FUNCTION F_SetStateParams : BOOL;
VAR_INPUT
    nStateRef    :    UDINT;
    rPosition    :    REAL;
    rTolerance: REAL;
    stBeamParams    :    ST_BeamParams;
END_VAR
VAR_IN_OUT
    Table    :    FB_LinearDeviceStateTable;
END_VAR
VAR
    stDeviceState    :    ST_DeviceState;
    
END_VAR

stDeviceState.nStateRef := nStateRef;
stDeviceState.rPosition := rPosition;
stDeviceState.rTolerance := rTolerance;
stDeviceState.stReqBeamParam := stBeamParams;

Table.A_Add(
    key := nStateRef,
    putValue := stDeviceState
);

F_SetStateParams := Table.bOk;

END_FUNCTION
